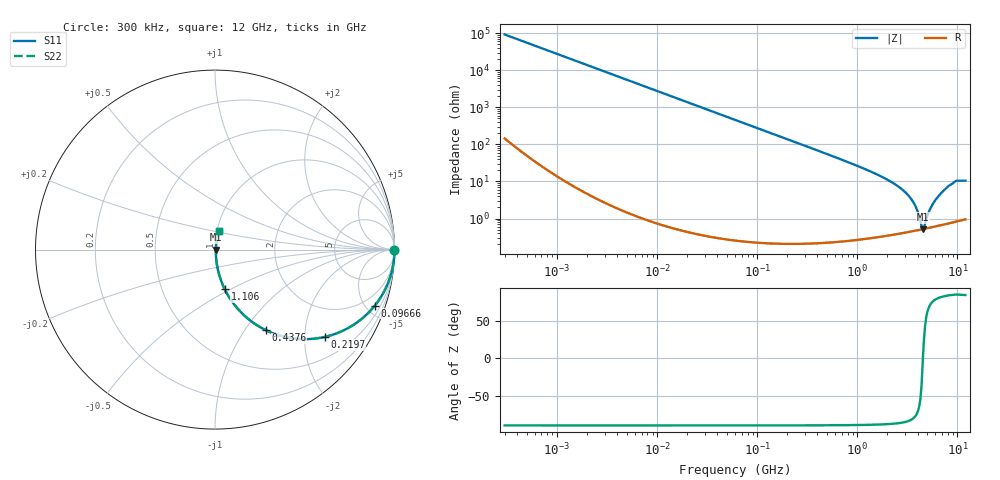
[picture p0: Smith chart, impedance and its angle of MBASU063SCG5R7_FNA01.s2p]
! MBASU063SCG5R7_FNA01  S-PARAMETER MODEL  ( General Type )
! Model Generated by TAIYO YUDEN Corporation (http://www.ty-top.com)
! Version 1.0
! TAIYO YUDEN Control No. 130801
! Copyright(c) 2013 TAIYO YUDEN CO.,LTD. All Rights Reserved.
! Product Description (link to TY-COMPAS)
! https://ds.yuden.co.jp/TYCOMPAS/or/detail?pn=MBASU063SCG5R7DFNA01&u=M
! Products Name : Multilayer Ceramic Capacitors
! Characteristics :
!  Capacitance : 5.7 pF , Rated Voltage : 50V , TCC : CG / C0G
!  Case Size : 0.6 x 0.3 / 0.024 x 0.012 [mm/inch] , Thickness : 0.3 / 0.012 [mm/inch]
!  (Conditions: Temperature = 25 degC , DC Bias Current/Voltage = 0A / 0V)
! External Node Assignments :
!  1  o---| |---o  2
! GND o---------o GND
! Frequency Range : 0.3MHz  -  12000MHz  [ 401 STEP ]
# MHz S RI R 50
! Freq[MHz].  S11 Real  S11 Imag  S21 Real  S21 Imag  S12 Real  S12 Imag  S22 Real  S22 Imag
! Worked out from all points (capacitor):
!   401 points, 300 kHz to 12 GHz, reference 50 ohm
!   read as one part in series: C = 5.76 pF near 316.3 kHz
!   lowest |Z| = 517 mohm at 4.503 GHz (marker M1)
!   series resonance near 4.516 GHz, so ESL is about 220 pH
!   S11 on the Smith chart (normalised r, x): 300 kHz: open; 96.66 MHz: 1.00, -5.72; 219.7 MHz: 1.00, -2.51; 437.6 MHz: 1.00, -1.25; 1.106 GHz: 1.01, -0.47; 12 GHz: 1.02, +0.21
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0.3  1 -0.00109  2.88e-06 0.00109  2.88e-06 0.00109  1 -0.00109
1.769972  1 -0.0064  4.32e-05 0.0064  4.32e-05 0.0064  1 -0.0064
10.44266  0.9986 -0.0377  0.00143 0.0377  0.00143 0.0377  0.9986 -0.0377
60  0.9549 -0.2072  0.0451 0.2072  0.0451 0.2072  0.9549 -0.2072
96.65937  0.8908 -0.3115  0.1092 0.3115  0.1092 0.3115  0.8908 -0.3115
219.7372  0.6116 -0.4866  0.3884 0.4866  0.3884 0.4866  0.6116 -0.4866
353.9943  0.3763 -0.4831  0.6237 0.4831  0.6237 0.4831  0.3763 -0.4831
437.5599  0.2822 -0.4483  0.7178 0.4483  0.7178 0.4483  0.2822 -0.4483
686.4755  0.1356 -0.3393  0.8644 0.3393  0.8644 0.3393  0.1356 -0.3393
1105.905  0.0547 -0.2216  0.9453 0.2216  0.9453 0.2216  0.0547 -0.2216
2088.533  0.0141 -0.1022  0.9859 0.1022  0.9859 0.1022  0.0141 -0.1022
2795.104  0.00766 -0.0603  0.9923 0.0603  0.9923 0.0603  0.00766 -0.0603
3364.605  0.00571 -0.0362  0.9943 0.0362  0.9943 0.0362  0.00571 -0.0362
3841.137  0.0051 -0.0197  0.9949 0.0197  0.9949 0.0197  0.0051 -0.0197
4270.516  0.00503 -0.00675  0.995 0.00675  0.995 0.00675  0.00503 -0.00675
4502.883  0.00513 -0.000292  0.9949 0.000292  0.9949 0.000292  0.00513 -0.000292
4747.894  0.00531 0.00497  0.9947 -0.00497  0.9947 -0.00497  0.00531 0.00497
5140.631  0.00571 0.0131  0.9943 -0.0131  0.9943 -0.0131  0.00571 0.0131
5565.855  0.00626 0.0215  0.9937 -0.0215  0.9937 -0.0215  0.00626 0.0215
6879.757  0.00884 0.0473  0.9912 -0.0473  0.9912 -0.0473  0.00884 0.0473
9454.42  0.0177 0.0974  0.9823 -0.0974  0.9823 -0.0974  0.0177 0.0974
12000  0.0199 0.1014  0.9801 -0.1014  0.9801 -0.1014  0.0199 0.1014
